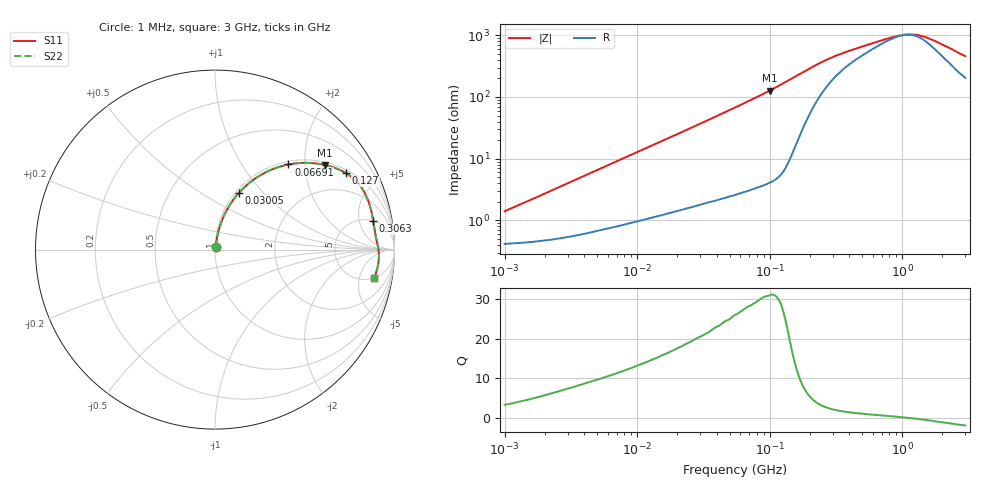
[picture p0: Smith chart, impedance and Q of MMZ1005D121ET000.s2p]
! S-parameter Generated by TDK Corporation
! Copyright(C) 2016 TDK Corporation.
! All Rights Reserved.
! TDK P/N: MMZ1005D121ET000 (Chip Beads)
! Property: |Z|=120¶ at 100MHz
! Size(LxWxT): 1x0.5x0.5mm, 0.039x0.02x0.02inches
! Model Type: s2p (Touchstone File Format Version 1.0)
! Frequency: DC=Yes Start=1MHz Stop=3000MHz 202points Log-sweep
! Note: This model was converted from impedance.
! Model Generated on May. 16, 2016
! Hash(MD5):
! Port Assignments:
!  1 ---@@@--- 2
! Applicable Conditions:
!  Temperature = 25 degC
!  DC Bias Current = 0 A
!  Small Signal Operation
! Terms and conditions regarding TDK Simulation Models
! (1)This simulation model is being provided solely for informational purposes. Please refer to the specifications of the products in terms of detailed characteristics of such products.
! (2)In no event shall TDK Corporation of any of its subsidiaries be liable for any loss or damage arising, directly or indirectly,
!  From any information contained in this simulation model, including, but not limited to loss or damages arising from any inaccuracies, omissions or errors in connection with such information.
! (3)Any and all copyrights on this simulation model are owned by TDK Corporation.
!  Duplication or redistribution of this simulation model without prior written permission from TDK Corporation is prohibited.
! (4)This simulation model is subject to any modification or change without any prior notice.
! (5)Neither TDK Corporation nor any of its subsidiaries shall make any warranty, express or implied,
!  Including but not limited to the correctness, implied warranties of merchantability and fitness for a particular purpose with respect to this simulation models.
! (6)The use of this simulation model shall be deemed to have consented to the terms and conditions hereof.
# MHz S MA R 50
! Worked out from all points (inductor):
!   201 points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, 1 MHz to 3 GHz, reference 50 ohm
!   read as one part in series: L = 214 nH near 1.041 MHz
!   highest Q = 31 at 99.85 MHz (marker M1), where L = 202 nH
!   self-resonance near 1.061 GHz
!   S11 on the Smith chart (normalised r, x): 1 MHz: 1.01, +0.03; 30.05 MHz: 1.04, +0.74; 66.91 MHz: 1.06, +1.65; 127 MHz: 1.12, +3.34; 306.3 MHz: 5.06, +8.09; 3 GHz: 5.09, -8.21
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1  0.01405 72.1  0.9958 -0.8  0.9958 -0.8  0.01405 72.1
3.900413  0.05117 80.4  0.9927 -2.9  0.9927 -2.9  0.05117 80.4
8.017732  0.1016 79.4  0.9864 -5.8  0.9864 -5.8  0.1016 79.4
14.61624  0.1787 76.0  0.9724 -10.3  0.9724 -10.3  0.1787 76.0
21.81181  0.2582 71.9  0.952 -14.9  0.952 -14.9  0.2582 71.9
30.0453  0.3426 67.2  0.923 -20.0  0.923 -20.0  0.3426 67.2
41.38676  0.4461 61.1  0.876 -26.5  0.876 -26.5  0.4461 61.1
54.77226  0.5495 54.5  0.8147 -33.3  0.8147 -33.3  0.5495 54.5
66.90963  0.6263 49.2  0.7575 -38.8  0.7575 -38.8  0.6263 49.2
81.73662  0.702 43.5  0.6889 -44.6  0.6889 -44.6  0.702 43.5
99.84923  0.7728 37.6  0.6103 -50.6  0.6103 -50.6  0.7728 37.6
126.9575  0.8444 30.3  0.5052 -57.5  0.5052 -57.5  0.8444 30.3
161.4254  0.885 23.3  0.3965 -61.9  0.3965 -61.9  0.885 23.3
213.6344  0.8968 16.3  0.2872 -61.0  0.2872 -61.0  0.8968 16.3
306.2963  0.8955 10.2  0.1979 -53.2  0.1979 -53.2  0.8955 10.2
457.0858  0.8965 6.2  0.1452 -41.5  0.1452 -41.5  0.8965 6.2
800.5644  0.9054 2.1  0.1006 -18.8  0.1006 -18.8  0.9054 2.1
939.5906  0.9087 0.9  0.09244 -8.8  0.09244 -8.8  0.9087 0.9
1059.487  0.9108 0.0  0.0892 -0.1  0.0892 -0.1  0.9108 0.0
1294.266  0.9138 -1.6  0.09011 16.2  0.09011 16.2  0.9138 -1.6
1645.649  0.9143 -3.7  0.1059 34.2  0.1059 34.2  0.9143 -3.7
3000  0.8973 -10.1  0.1956 53.4  0.1956 53.4  0.8973 -10.1
